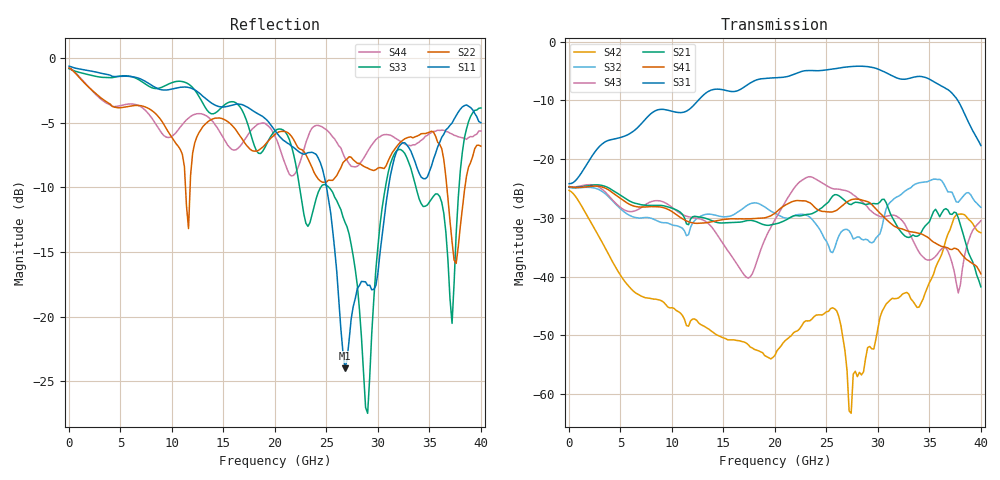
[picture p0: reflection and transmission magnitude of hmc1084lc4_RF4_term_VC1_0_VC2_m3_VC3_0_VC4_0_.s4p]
!Agilent Technologies,N5224A,MY51441122,A.09.40.06
!Agilent N5224A: A.09.40.06
!Date: Thursday, June 19, 2014 00:54:38
!Correction: S11(Full 4 Port(1,2,3,4))
!S12(Full 4 Port(1,2,3,4))
!S13(Full 4 Port(1,2,3,4))
!S14(Full 4 Port(1,2,3,4))
!S21(Full 4 Port(1,2,3,4))
!S22(Full 4 Port(1,2,3,4))
!S23(Full 4 Port(1,2,3,4))
!S24(Full 4 Port(1,2,3,4))
!S31(Full 4 Port(1,2,3,4))
!S32(Full 4 Port(1,2,3,4))
!S33(Full 4 Port(1,2,3,4))
!S34(Full 4 Port(1,2,3,4))
!S41(Full 4 Port(1,2,3,4))
!S42(Full 4 Port(1,2,3,4))
!S43(Full 4 Port(1,2,3,4))
!S44(Full 4 Port(1,2,3,4))
!S4P File: Measurements: <S11,S12,S13,S14>,
!<S21,S22,S23,S24>,
!<S31,S32,S33,S34>,
!<S41,S42,S43,S44>:
# Hz S  dB  R 50
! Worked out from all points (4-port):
!   201 points, 10 MHz to 40 GHz, reference 50 ohm
!   strongest paths, dB at 10 MHz, 10.01 GHz, 20 GHz, 30 GHz, 40 GHz:
!     S31: -24.2, -11.9, -6.2, -4.7, -17.7
!     S41: -24.7, -28.9, -29.2, -28.9, -39.5
!     S21: -24.8, -28.4, -31.1, -27.6, -41.8
!     S43: -24.8, -28.2, -30.3, -29.6, -30.5
!     S32: -24.8, -31.2, -29.2, -33.1, -28.2
!     S42: -25.3, -45.3, -53.4, -48.8, -32.5
!   lowest |S11| = -24.0 dB at 26.8 GHz (marker M1), VSWR 1.13, Z = 50 + j6.32 ohm
!   |S11| at or under -10 dB: 25.01 GHz to 31.02 GHz (6.007 GHz wide, 21.4 % of centre)
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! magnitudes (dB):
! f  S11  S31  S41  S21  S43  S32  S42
! 10 MHz  -0.6  -24.2  -24.7  -24.8  -24.8  -24.8  -25.3
! 17.41 GHz  -3.8  -7.3  -30.2  -30.4  -40.3  -27.8  -51.6
! 26.8 GHz  -24.0  -4.3  -27.5  -27.1  -25.3  -32.0  -52.7
! 29 GHz  -17.6  -4.2  -27.3  -27.7  -28.2  -33.8  -52.1
! 31.4 GHz  -8.4  -5.8  -31.2  -30.0  -29.6  -27.0  -43.7
! 37.2 GHz  -5.0  -8.8  -35.4  -29.4  -37.7  -25.6  -31.0
! 40 GHz  -5.0  -17.7  -39.5  -41.8  -30.5  -28.2  -32.5
